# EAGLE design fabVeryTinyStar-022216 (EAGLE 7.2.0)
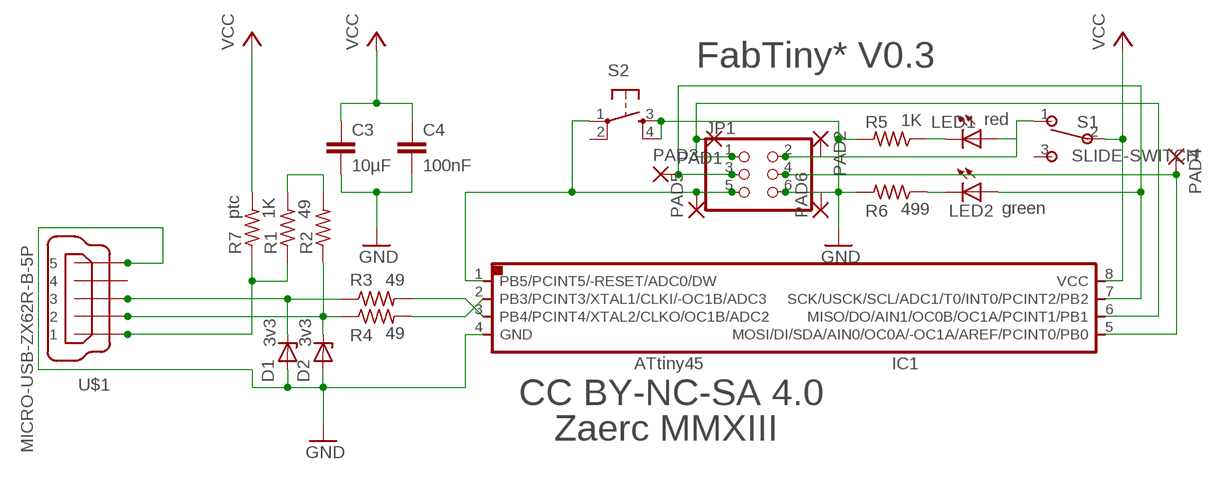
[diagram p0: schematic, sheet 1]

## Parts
C3  10µF  C-EUC0603  [C0603]
C4  100nF  C-EUC0603  [C0603]
D1  3v3  ZENER_DIODESOD123  [SOD123]
D2  3v3  ZENER_DIODESOD123  [SOD123]
IC1  ATTINY*5  ATTINY45SI  [SOIC8]
JP1  PINHD-2X3_2.54-SMD  [2X03SMD]
LED1  red  LEDCHIPLED_0603  [CHIPLED_0603]
LED2  green  LEDCHIPLED_0603  [CHIPLED_0603]
PAD1  SMD2  [SMD1,27-2,54]
PAD2  SMD2  [SMD1,27-2,54]
PAD3  SMD2  [SMD1,27-2,54]
PAD4  SMD2  [SMD1,27-2,54]
PAD5  SMD2  [SMD1,27-2,54]
PAD6  SMD2  [SMD1,27-2,54]
R1  1K  RESISTOR0402  [0402]
R2  49  RESISTOR0402  [0402]
R3  49  RESISTOR0402  [0402]
R4  49  RESISTOR0402  [0402]
R5  1K  RESISTOR0402  [0402]
R6  499  RESISTOR0402  [0402]
R7  ptc  RESISTOR1206  [1206]
S1  SLIDE-SWITCH  [AYZ0102AGRLC]
S2  6MM_SWITCH6MM_SWITCH  [6MM_SWITCH]
U$1  MICRO-USB-ZX62R-B-5P  [ZX62R-B-5P]

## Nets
5V: R1.1 R7.1 U$1.1
B0: IC1.5(MOSI/DI/SDA/AIN0/OC0A/-OC1A/AREF/PCINT0/PB0) JP1.4 PAD4.1(P)
B1: IC1.6(MISO/DO/AIN1/OC0B/OC1A/PCINT1/PB1) JP1.1 PAD1.1(P)
B2: IC1.7(SCK/USCK/SCL/ADC1/T0/INT0/PCINT2/PB2) JP1.3 LED2.A PAD3.1(P)
B3: IC1.2(PB3/PCINT3/XTAL1/CLKI/-OC1B/ADC3) R4.2
B4: IC1.3(PB4/PCINT4/XTAL2/CLKO/OC1B/ADC2) R3.2
B5: IC1.1(PB5/PCINT5/-RESET/ADC0/DW) JP1.5 PAD5.1(P) S2.1(P)
D+: D1.CATHODE R3.1 U$1.3
D-: D2.CATHODE R2.1 R4.1 U$1.2
GND: C3.2 C4.2 D1.ANODE D2.ANODE IC1.4(GND) JP1.6 PAD6.1(P) R5.2 R6.2 S2.3(S) S2.4(S1) U$1.5
N$1: R1.2 R2.2
N$13: LED2.C R6.1
N$14: LED1.C R5.1
TP: JP1.2 LED1.A PAD2.1(P) S1.1
VCC: C3.1 C4.1 IC1.8(VCC) R7.2 S1.2
Unconnected: S1.3 S2.2(P1) U$1.4

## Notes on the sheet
- FabTiny* V0.3
- CC BY-NC-SA 4.0
- Zaerc MMXIII

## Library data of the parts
C3 C4 = rcl:C-EU: CAPACITOR, European symbol
D1 D2 = 01_fab:ZENER_DIODE: zener diode
IC1 = 01_fab:ATTINY45
JP1 = pinhead:PINHD-2X3: PIN HEADER
LED1 LED2 = led:LED: LED
PAD1-PAD6 = wirepad:SMD2: SMD PAD
R1-R7 = 01_FAB_Hello:RESISTOR
S1 = Zaerc:SLIDE-SWITCH
S2 = 01_fab:6MM_SWITCH: OMRON SWITCH
U$1 = con-hirose:MICRO-USB-: Hirose Micro USB Connector ZX62R-B-5P: Micro B, reverse (top mount) shell SMT Supplier: DigiKey H11574CT-ND Source: http://www.hirose.co.jp/cataloge_hp/e24200011.pdf

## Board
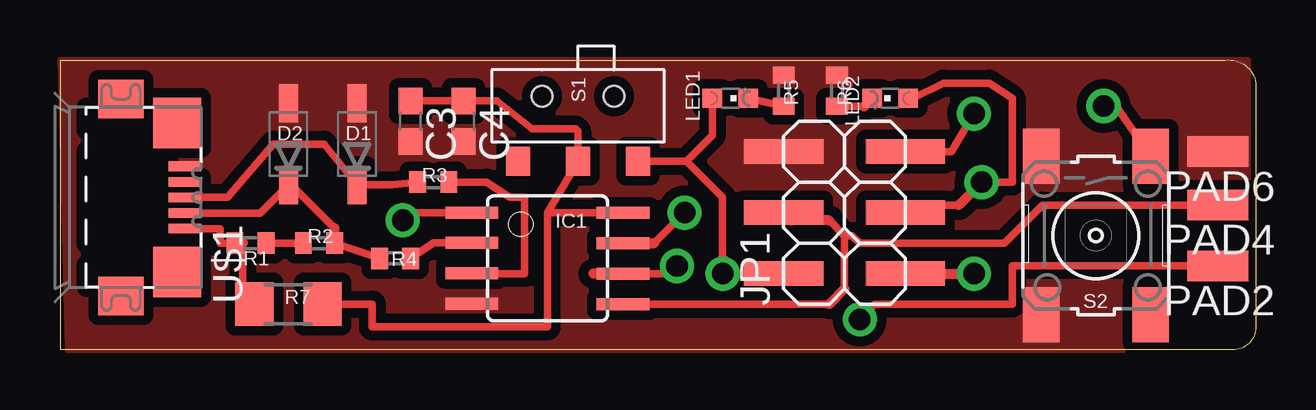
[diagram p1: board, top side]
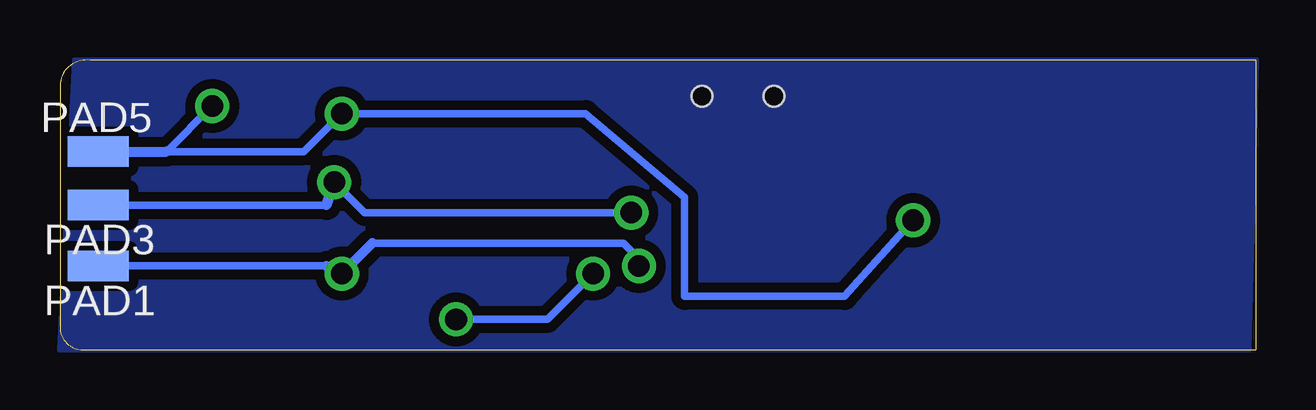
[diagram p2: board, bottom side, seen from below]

Size 49.85 x 12.08 mm. Coordinates in mm from the lower left corner, seen from the top.
Outline: 0,12.06 48.58,12.06 arc-90 49.85,11.11 49.85,0.95 arc-90 48.9,0 0,0 0,12.06
Copper layers (1*16): Top 0.035mm / dielectric 1.5mm / Bottom 0.035mm
Design rules "default *": minimum track width 10mil, minimum drill 24mil, track to track 16mil, track to pad 16mil, pad to pad 16mil, via to via 16mil, smd to smd 8mil, copper to edge 0mil, drill to drill 8mil, minimum pad ring 10mil, minimum via ring 8mil, stop-mask expansion 4mil, vias tented up to drill 0mil, thermal gap 10mil

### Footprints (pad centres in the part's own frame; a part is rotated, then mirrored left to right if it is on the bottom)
C0603 = smd 1.1 x 1: 1 -0.85,0; 2 0.85,0
SOD123 = smd 1.6 x 0.8: ANODE 1.7,0; CATHODE -1.7,0
SOIC8 = smd 0.5 x 2.2: 1 -1.905,-3.154; 2 -0.645,-3.154; 3 0.625,-3.154; 4 1.895,-3.154; 5 1.905,3.154; 6 0.635,3.154; 7 -0.635,3.154; 8 -1.905,3.154
2X03SMD = smd 1.016 x 3.302: 1 -1.27,-3.81; 2 -1.27,1.27; 3 1.27,-3.81; 4 1.27,1.27; 5 3.81,-3.81; 6 3.81,1.27
CHIPLED_0603 = smd 0.8 x 0.8: A 0,-0.75; C 0,0.75
SMD1,27-2,54 = smd 1.27 x 2.54: 1 0,0
0402 = smd 0.7 x 0.9: 1 -0.65,0; 2 0.65,0
1206 = smd 1.6 x 1.803: 1 -1.422,0; 2 1.422,0
AYZ0102AGRLC = smd 1 x 1.2: 1 2.5,-2.3; 2 0,-2.3; 3 -2.5,-2.3 | hole 0.85: -1.5,0.4; 1.5,0.4
6MM_SWITCH = smd 2.286 x 1.524: 1 -3.302,2.286; 2 3.302,2.286; 3 -3.302,-2.286; 4 3.302,-2.286
ZX62R-B-5P = smd 1.35 x 0.4: 1 2.675,-1.3; 2 2.675,-0.65; 3 2.675,0; 4 2.675,0.65; 5 2.675,1.3 | smd 1.9 x 1.6: M1 0,-4.1; M2 0,4.1 | smd 2 x 2.1: M3 2.35,3.1; M4 2.35,-3.1

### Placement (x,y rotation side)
C3  14.61,9.53 270 top
C4  16.83,9.53 270 top
D1  12.38,8.57 90 top
D2  9.53,8.57 90 top
IC1  20.32,3.81 270 top
JP1  31.43,4.45 90 top
LED1  27.94,10.48 270 top
LED2  34.61,10.48 90 top
PAD1  48.26,3.49 90 bottom
PAD2  48.26,3.49 90 top
PAD3  48.26,6.03 90 bottom
PAD4  48.26,6.03 90 top
PAD5  48.26,8.25 270 bottom
PAD6  48.26,8.25 90 top
R1  7.94,4.45 0 top
R2  10.79,4.45 180 top
R3  15.56,6.98 0 top
R4  13.97,3.81 0 top
R5  30.16,10.79 90 top
R6  32.38,10.79 90 top
R7  9.53,1.91 0 top
S1  21.59,10.16 0 top
S2  43.18,4.76 270 top
U$1  2.54,6.35 0 top

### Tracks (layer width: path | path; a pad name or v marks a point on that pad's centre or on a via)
5V
  Top 0.305: U$1.1 6.67,5.05 6.67,4.44 R1.1 | 7.62,4.44 7.62,1.91
  Top 0.406: 7.62,4.44 R1.1 | 7.62,1.91 R7.1
B0
  Top 0.305: IC1.5 32.07,1.91 | 32.7,2.54 32.7,4.76 | 32.7,4.76 32.07,5.4 | 32.7,4.76 33.02,4.76 33.34,4.44 39.37,4.44 40.96,6.03 PAD4.1
  Top 0.406: 32.07,1.91 32.7,2.54 | 32.07,5.4 30.48,5.4 JP1.4
B1  (via drill 0.9 pad 1.42)
  Top 0.305: IC1.6 25.72,3.18
  Top 0.406: IC1.6 22.22,3.18 | 25.72,3.18 v25.72,3.49 | JP1.1 v38.1,3.18
  Bottom 0.305: PAD1.1 38.74,3.49 | 25.72,3.81 26.35,4.44 36.83,4.44
  Bottom 0.406: 38.74,3.49 v38.1,3.18 36.83,4.44 | v25.72,3.49 25.72,3.81
B2  (via drill 0.9 pad 1.42)
  Top 0.305: 24.77,4.44 v26.04,5.72 | v38.42,6.98 39.69,6.98 39.69,10.48 38.74,11.11 36.83,11.11 35.56,10.48 | 37.47,6.03 35.56,6.03
  Top 0.406: IC1.7 24.77,4.44 | LED2.A 35.56,10.48 | v38.42,6.98 37.47,6.03 | 35.56,6.03 JP1.3
  Bottom 0.305: PAD3.1 38.74,6.03 | v26.04,5.72 37.15,5.72 v38.42,6.98
  Bottom 0.406: 38.74,6.03 v38.42,6.98
B3
  Top 0.305: IC1.2 15.58,4.46 R4.2
B4
  Top 0.305: R3.2 17.78,6.98 18.73,6.35 19.37,6.35 19.37,3.18 17.81,3.18
  Top 0.406: 17.81,3.18 IC1.3
B5  (via drill 0.9 pad 1.42)
  Top 0.305: IC1.1 14.61,5.72 v14.29,5.4 | v38.1,9.84 37.15,8.25 JP1.5 | 44.01,10.16 S2.1
  Top 0.406: v43.5,10.16 44.01,10.16
  Bottom 0.305: v14.29,5.4 17.14,2.22 23.81,2.22 23.81,6.35 27.94,9.84 v38.1,9.84 39.69,8.25 PAD5.1 | 45.4,8.25 v43.5,10.16
  Bottom 0.406: PAD5.1 45.4,8.25
D+
  Top 0.305: U$1.3 6.98,6.35 8.89,8.57 11,8.57 D1.CATHODE 13.84,6.87 R3.1
D-
  Top 0.305: R2.1 R4.1 | U$1.2 8.35,5.7 D2.CATHODE | 9.64,6.87 11.43,5.08
  Top 0.406: D2.CATHODE 9.64,6.87 | 11.43,5.08 11.43,4.46 R2.1
GND
  pour Top (isolate 0.406, rank 6, no thermals): 0.32,0 49.53,0 49.53,12.06 0,12.06
  pour Bottom: 0.32,0 49.85,0 49.21,12.06 0,12.06
N$1
  Top 0.305: R1.2 R2.2
N$13
  Top 0.305: R6.1 33.53,10.14
  Top 0.406: 33.53,10.14 LED2.C
N$14
  Top 0.305: LED1.C R5.1
TP  (via drill 0.9 pad 1.42)
  Top 0.305: S1.1 26.11,7.86 | 26.11,7.86 27.62,6.35 27.62,3.81 | LED1.A 27.19,8.94 26.11,7.86 | PAD2.1 39.69,3.49 39.69,1.91 33.97,1.91 v33.34,1.27
  Top 0.406: JP1.2 28.26,3.18 27.62,3.81 v27.62,3.18
  Bottom 0.305: v33.34,1.27 29.53,1.27 v27.62,3.18
VCC
  Top 0.305: R7.2 13.02,1.91 13.02,0.95 20.32,0.95 20.32,5.72 | 20.32,5.72 IC1.8 | 20.32,5.72 S1.2 21.59,9.11 21.49,9.21 19.68,9.21 18.2,10.38 C4.1 C3.1

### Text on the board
bDocu: FabVeryTiny* v0.1 | CC BY-NC-SA 4.0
